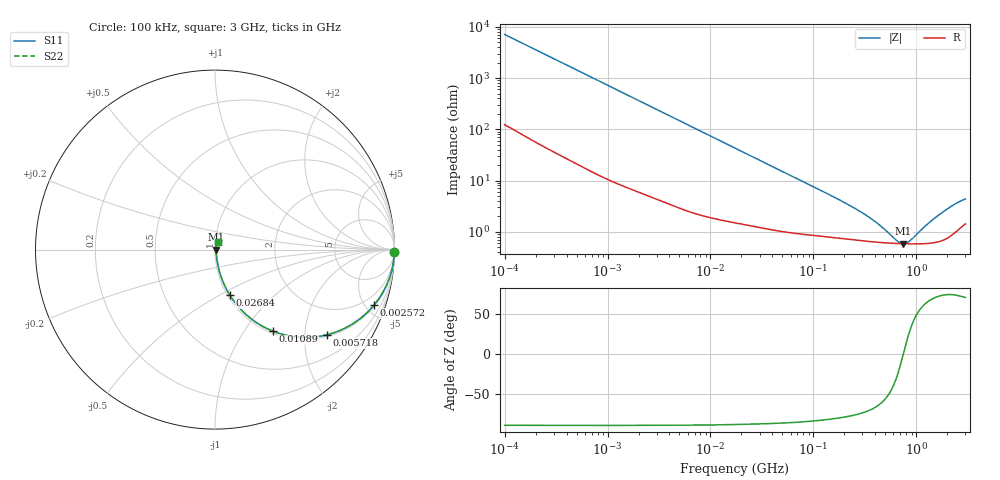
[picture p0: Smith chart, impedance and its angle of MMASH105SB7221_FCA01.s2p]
! MMASH105SB7221_FCA01  S-PARAMETER MODEL  ( Standard Model )
! Model Generated by TAIYO YUDEN Corporation (http://www.ty-top.com)
! Version 1.0
! TAIYO YUDEN Control No. 220601
! Copyright(c) 2019 TAIYO YUDEN CO.,LTD. All Rights Reserved.
! Product Description (link to TY-COMPAS)
! https://ds.yuden.co.jp/TYCOMPAS/or/detail?pn=MMASH105SB7221KFCA01&u=M
! Products Name : Multilayer Ceramic Capacitors
! Characteristics :
!  Capacitance : 220 [pF] , Rated Voltage : 100 [V] , TCC : X7R
!  Case Size : 1.0 x 0.5 / 0.039 x 0.02 [mm/inch] , Thickness : 0.5 / 0.02 [mm/inch]
!  (Conditions: Temperature = 25 [degC] , DC Bias Voltage = 0 [V])
! External Node Assignments :
!  1  o---| |---o  2
! GND o---------o GND
! Frequency Range : 100kHz  -  3GHz  [ 401 STEP ]
# MHZ S RI R 50
! Freq[MHz].  S11 Real  S11 Imag  S21 Real  S21 Imag  S12 Real  S12 Imag  S22 Real  S22 Imag
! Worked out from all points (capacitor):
!   401 points, 100 kHz to 3 GHz, reference 50 ohm
!   read as one part in series: C = 223 pF near 105.3 kHz
!   lowest |Z| = 582 mohm at 746 MHz (marker M1)
!   series resonance near 747.5 MHz, so ESL is about 200 pH
!   S11 on the Smith chart (normalised r, x): 100 kHz: open; 2.572 MHz: 1.10, -5.70; 5.718 MHz: 1.05, -2.58; 10.89 MHz: 1.04, -1.36; 26.84 MHz: 1.03, -0.56; 3 GHz: 1.03, +0.08
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0.1  0.9996 -0.014  0.00044 0.014  0.00044 0.014  0.9996 -0.014
0.562235  0.9929 -0.077  0.00709 0.077  0.00709 0.077  0.9929 -0.077
1.218153  0.9706 -0.1618  0.0294 0.1618  0.0294 0.1618  0.9706 -0.1618
2.572132  0.8864 -0.309  0.1136 0.309  0.1136 0.309  0.8864 -0.309
3.161081  0.8395 -0.3583  0.1605 0.3583  0.1605 0.3583  0.8395 -0.3583
5.718342  0.623 -0.4746  0.377 0.4746  0.377 0.4746  0.623 -0.4746
7.79083  0.4753 -0.4883  0.5247 0.4883  0.5247 0.4883  0.4753 -0.4883
10.89156  0.3218 -0.4541  0.6782 0.4541  0.6782 0.4541  0.3218 -0.4541
17.7727  0.1586 -0.3481  0.8414 0.3481  0.8414 0.3481  0.1586 -0.3481
26.84345  0.0823 -0.2532  0.9177 0.2532  0.9177 0.2532  0.0823 -0.2532
49.82709  0.0318 -0.1453  0.9682 0.1453  0.9682 0.1453  0.0318 -0.1453
97.38194  0.0143 -0.0758  0.9857 0.0758  0.9857 0.0758  0.0143 -0.0758
294.964  0.00713 -0.0225  0.9929 0.0225  0.9929 0.0225  0.00713 -0.0225
412.3589  0.00638 -0.0135  0.9936 0.0135  0.9936 0.0135  0.00638 -0.0135
547.5153  0.006 -0.00682  0.994 0.00682  0.994 0.00682  0.006 -0.00682
655.7614  0.00585 -0.00284  0.9941 0.00284  0.9941 0.00284  0.00585 -0.00284
745.9503  0.00579 -4.47e-05  0.9942 4.47e-05  0.9942 4.47e-05  0.00579 -4.47e-05
870.6963  0.00576 0.00335  0.9942 -0.00335  0.9942 -0.00335  0.00576 0.00335
1281.618  0.00601 0.0126  0.994 -0.0126  0.994 -0.0126  0.00601 0.0126
1838.476  0.00737 0.0234  0.9926 -0.0234  0.9926 -0.0234  0.00737 0.0234
2441.062  0.0111 0.0337  0.9889 -0.0337  0.9889 -0.0337  0.0111 0.0337
3000  0.0156 0.0399  0.9844 -0.0399  0.9844 -0.0399  0.0156 0.0399
